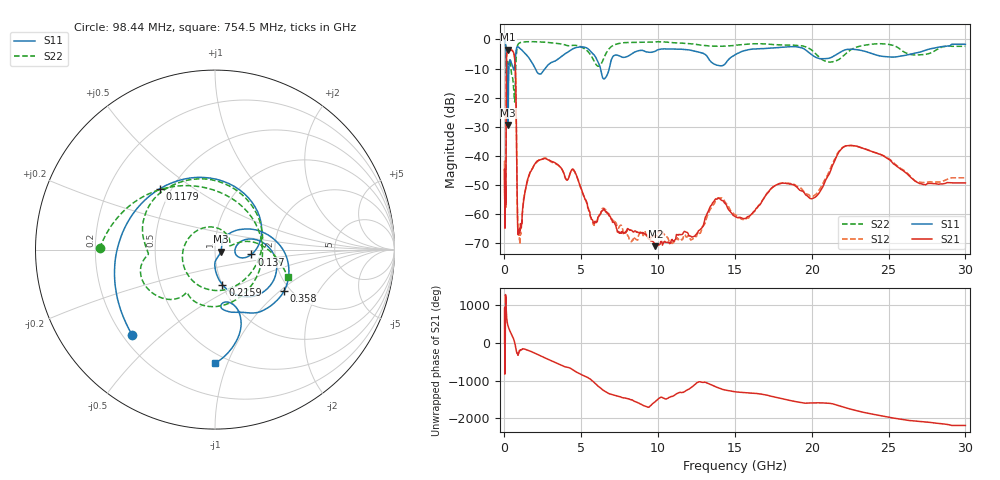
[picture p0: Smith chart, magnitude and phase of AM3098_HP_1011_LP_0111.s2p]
! Date/Time: Thu, Feb 28, 2019 8:43 AM
! Network Analyzer: Agilent Technologies E8364B Rev: A.07.50.67
! Sweep from 0.010 to 30.000 GHz, 1601 Points, Sweep Type: LOG
! Power Supply: 5.022 V, 0.002 A
# Hz S DB R 50
!freq MagS11 AngS11 MagS21 AngS21 MagS12 AngS12 MagS22 AngS22
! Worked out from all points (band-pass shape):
!   1601 points, 10 MHz to 30 GHz, reference 50 ohm
!   highest |S21| = -3.49 dB at 238.7 MHz (marker M1); lowest = -71.0 dB at 9.829 GHz (marker M2)
!   |S21| within 3 dB of the highest: 136.6 MHz to 665.7 MHz (529.1 MHz wide, 132 % of centre)
!   lowest |S11| = -29.3 dB at 239.9 MHz (marker M3), VSWR 1.07, Z = 53.3 - j1.14 ohm
!   |S11| at or under -10 dB: 200.6 MHz to 290.7 MHz (90.14 MHz wide, 36.7 % of centre); 2.009 GHz to 2.646 GHz (637.4 MHz wide, 27.4 % of centre); 6.251 GHz to 6.823 GHz (571.8 MHz wide, 8.75 % of centre)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
!   |S22| runs from -21.5 to -0.5 dB; largest |S21 - S12| = 0.012
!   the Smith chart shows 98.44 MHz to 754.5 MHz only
!   S11 on the Smith chart (normalised r, x): 98.44 MHz: 0.24, -0.40; 117.9 MHz: 0.43, +0.37; 137 MHz: 1.51, -0.08; 215.9 MHz: 1.00, -0.41; 358 MHz: 1.86, -1.07; 754.5 MHz: 0.43, -0.90
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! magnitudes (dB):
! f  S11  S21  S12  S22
! 10 MHz  -0.3  -44.7  -44.8  -0.5
! 38.04 MHz  -0.4  -62.6  -60.8  -0.8
! 98.44 MHz  -3.6  -50.5  -51.1  -3.8
! 117.9 MHz  -6.8  -20.7  -20.7  -10.9
! 137 MHz  -13.8  -6.4  -6.4  -10.4
! 144.7 MHz  -18.5  -5.2  -5.2  -10.9
! 215.9 MHz  -14.0  -3.7  -3.6  -8.1
! 238.7 MHz  -29.3  -3.5  -3.5  -8.6
! 239.9 MHz  -29.3  -3.5  -3.5  -8.6
! 358 MHz  -7.0  -3.8  -3.8  -7.5
! 550.5 MHz  -9.5  -4.1  -4.1  -13.9
! 662.4 MHz  -9.5  -6.3  -6.3  -21.5
! 754.5 MHz  -4.0  -20.9  -20.9  -7.3
! 859.3 MHz  -2.5  -64.1  -62.3  -1.9
! 978.7 MHz  -2.9  -66.3  -68.9  -1.2
! 2.084 GHz  -10.8  -42.0  -42.3  -0.8
! 4.503 GHz  -3.1  -44.8  -45.1  -2.0
! 7.926 GHz  -6.0  -65.8  -66.2  -1.0
! 9.829 GHz  -4.0  -71.0  -67.3  -0.8
! 20 GHz  -5.2  -54.8  -53.8  -3.6
! 22.67 GHz  -3.4  -36.5  -36.5  -3.2
! 30 GHz  -1.6  -49.3  -47.5  -2.3
